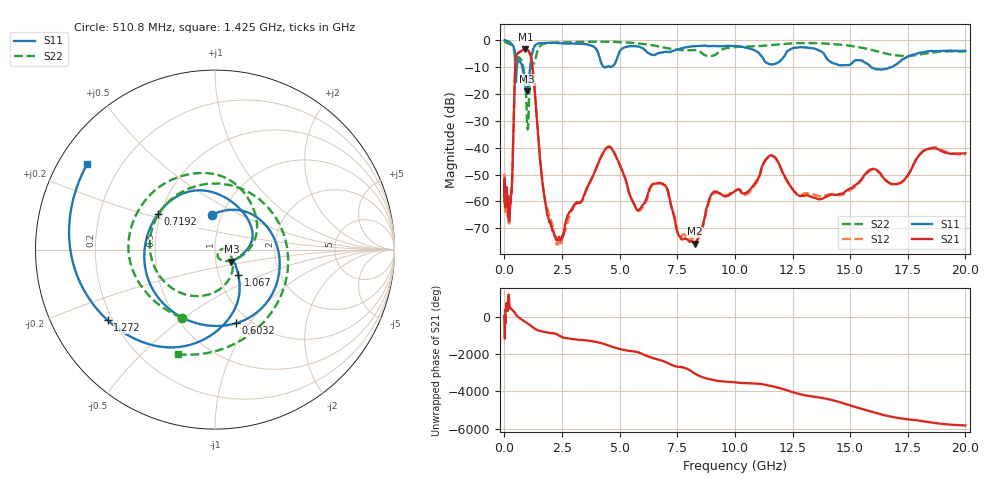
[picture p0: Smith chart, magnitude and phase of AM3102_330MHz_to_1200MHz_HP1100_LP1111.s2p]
! Date/Time: Tue, Sep 11, 2018 5:21 PM
! Network Analyzer: Agilent Technologies E8362B Rev: A.07.50.63
! Sweep from 0.010 to 20.000 GHz, 1601 Points, Sweep Type: LOG
! Power Supply: 4.949 V, 0.001 A
# Hz S DB R 50
!freq MagS11 AngS11 MagS21 AngS21 MagS12 AngS12 MagS22 AngS22
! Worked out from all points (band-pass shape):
!   1601 points, 10 MHz to 20 GHz, reference 50 ohm
!   highest |S21| = -3.21 dB at 916.3 MHz (marker M1); lowest = -75.8 dB at 8.266 GHz (marker M2)
!   |S21| within 3 dB of the highest: 501.5 MHz to 1.146 GHz (645 MHz wide, 78.3 % of centre)
!   lowest |S11| = -18.9 dB at 960.9 MHz (marker M3), VSWR 1.25, Z = 59.4 - j8.09 ohm
!   |S11| at or under -10 dB: 470.7 MHz to 538.4 MHz (67.68 MHz wide, 13.4 % of centre); 780.1 MHz to 1.118 GHz (338.4 MHz wide, 35.6 % of centre); 15.91 GHz to 16.77 GHz (857.2 MHz wide, 5.25 % of centre)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
!   |S22| runs from -33.2 to -0.2 dB; largest |S21 - S12| = 0.0092
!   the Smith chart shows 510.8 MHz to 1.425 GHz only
!   S11 on the Smith chart (normalised r, x): 510.8 MHz: 0.90, +0.36; 603.2 MHz: 0.86, -0.87; 719.2 MHz: 0.48, +0.22; 1.067 GHz: 1.24, -0.37; 1.272 GHz: 0.18, -0.29; 1.425 GHz: 0.08, +0.30
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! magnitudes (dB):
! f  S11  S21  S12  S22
! 10 MHz  -0.1  -51.7  -49.7  -0.2
! 35.55 MHz  -0.1  -58.1  -59.4  -0.5
! 126.4 MHz  -0.3  -59.0  -59.4  -1.1
! 317.7 MHz  -1.5  -55.6  -56.0  -1.9
! 447.2 MHz  -4.6  -15.5  -15.5  -4.6
! 510.8 MHz  -14.2  -5.7  -5.8  -7.5
! 603.2 MHz  -7.4  -4.7  -4.8  -6.3
! 719.2 MHz  -8.5  -4.0  -4.1  -7.1
! 916.3 MHz  -17.5  -3.2  -3.3  -17.2
! 960.9 MHz  -18.9  -3.3  -3.4  -23.9
! 1.067 GHz  -14.3  -4.2  -4.3  -22.5
! 1.272 GHz  -2.9  -14.3  -14.4  -8.7
! 1.425 GHz  -1.3  -31.4  -31.6  -4.2
! 1.59 GHz  -1.1  -48.1  -47.9  -1.8
! 2.325 GHz  -1.0  -74.4  -75.9  -0.8
! 4.457 GHz  -9.9  -40.0  -39.8  -0.5
! 5.652 GHz  -2.2  -61.6  -61.5  -1.0
! 6.803 GHz  -4.6  -53.2  -53.5  -2.5
! 8.266 GHz  -2.2  -75.8  -74.9  -3.6
! 11.53 GHz  -9.0  -42.9  -43.2  -1.8
! 13.74 GHz  -4.1  -59.1  -58.2  -1.1
! 20 GHz  -3.9  -42.1  -42.7  -4.1
